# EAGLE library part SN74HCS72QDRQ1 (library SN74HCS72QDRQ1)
Flip-Flops Automotive Schmitt-trigger input dual D-type negative-edge-triggered flip-flops w/ clear and preset 14-SOIC -40 to 125 Source: Datasheet
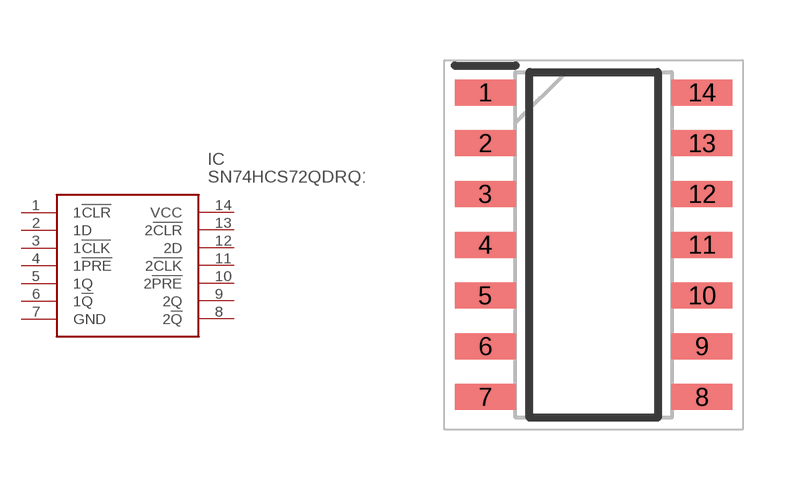
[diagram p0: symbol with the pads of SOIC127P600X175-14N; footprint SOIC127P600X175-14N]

Designator prefix IC

## SN74HCS72QDRQ1 (Arrow_Part_Number: SN74HCS72QDRQ1; Arrow_Price-Stock: https://www.arrow.com/en/products/sn74hcs72qdrq1/texas-instruments?region=nac; Description: Flip-Flops Automotive Schmitt-trigger input dual D-type negative-edge-triggered flip-flops w/ clear and preset 14-SOIC -40 to 125; Height: 1.75mm; Manufacturer_Name: Texas Instruments; Manufacturer_Part_Number: SN74HCS72QDRQ1; Mouser_Part_Number: 595-SN74HCS72QDRQ1; Mouser_Price-Stock: https://www.mouser.co.uk/ProductDetail/Texas-Instruments/SN74HCS72QDRQ1?qs=Cb2nCFKsA8rdYGfO8j6PMA%3D%3D)  [SOIC127P600X175-14N]
1  1!CLR
2  1D
3  1!CLK
4  1!PRE
5  1Q
6  1!Q
7  GND
8  2!Q
9  2Q
10  2!PRE
11  2!CLK
12  2D
13  2!CLR
14  VCC

## Footprint SOIC127P600X175-14N (pad centres in mm)
D
smd 1.525 x 0.65: 1 -2.712,3.81; 2 -2.712,2.54; 3 -2.712,1.27; 4 -2.712,0; 5 -2.712,-1.27; 6 -2.712,-2.54; 7 -2.712,-3.81; 8 2.712,-3.81; 9 2.712,-2.54; 10 2.712,-1.27; 11 2.712,0; 12 2.712,1.27; 13 2.712,2.54; 14 2.712,3.81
